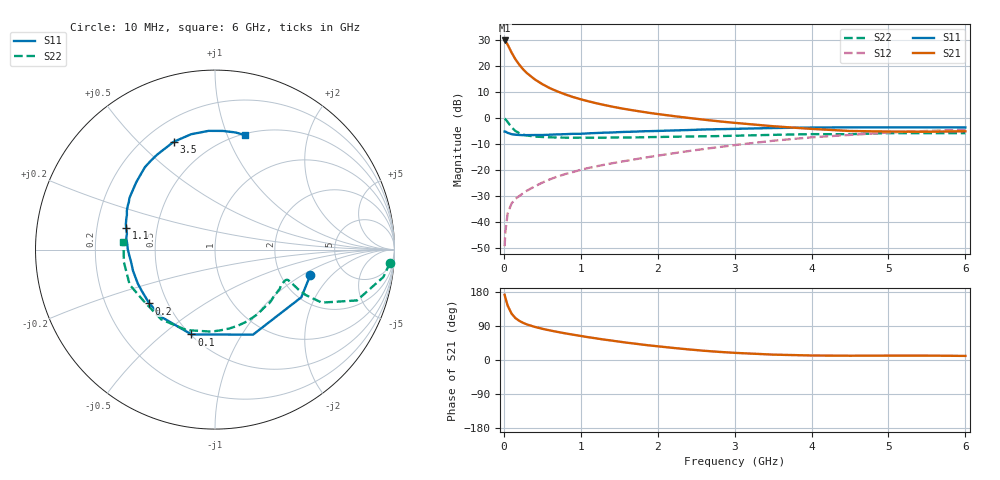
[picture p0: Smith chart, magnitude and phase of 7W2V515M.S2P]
! Infineon Technologies  Discrete & RF Semiconductors
! BFS17W
! Si NPN RF Bipolar Junction Transistor in SOT323
! VCE = 2.5 V  IC = 15 mA
! Common Emitter S-Parameters:  August  1999
# GHz  S  MA  R  50
!  f  S11  S21  S12  S22
! GHz  MAG  ANG  MAG  ANG  MAG  ANG  MAG  ANG
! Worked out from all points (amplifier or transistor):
!   36 points, 10 MHz to 6 GHz, reference 50 ohm
!   highest |S21| = 29.7 dB at 10 MHz (marker M1)
!   |S21| within 3 dB of that: start of sweep to 73.31 MHz
!   unconditionally stable (mu >= 1): 307.3 MHz to 2.534 GHz; 4.292 GHz to end of sweep
!   at 250 MHz: K = 0.93, MSG = 23.8 dB, |S12| = -28.8 dB
!   at 1.4 GHz: K = 1.21, MAG = 8.1 dB, |S12| = -17.4 dB
!   at 6 GHz: K = 1.08, MAG = -2.0 dB, |S12| = -4.4 dB
!   S11 on the Smith chart (normalised r, x): 10 MHz: 2.92, -1.18; 100 MHz: 0.51, -0.63; 200 MHz: 0.40, -0.31; 1.1 GHz: 0.33, +0.11; 3.5 GHz: 0.31, +0.64; 6 GHz: 0.52, +1.16
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0.01  0.55 -14.8  30.64 172.1  0.0035 81.5  0.9777 -4.3
0.02  0.5494 -28.9  29.83 163.8  0.0067 74.7  0.9499 -9.3
0.05  0.519 -65.9  25.45 143.4  0.0149 67.0  0.8401 -19.7
0.1  0.4906 -105.5  18.07 122.6  0.023 56.5  0.6644 -26.4
0.15  0.4788 -127.8  13.41 110.7  0.0283 54.8  0.565 -26.6
0.2  0.4733 -140.7  10.54 103.4  0.0319 56.8  0.5126 -25.5
0.25  0.4685 -149.9  8.61 98.1  0.0361 57.9  0.4804 -24.2
0.3  0.47 -156.2  7.264 93.9  0.0405 59.9  0.4634 -23.4
0.4  0.4718 -165.5  5.531 87.5  0.0488 62.2  0.4411 -22.6
0.5  0.4726 -171.7  4.458 82.4  0.0578 64.6  0.433 -22.8
0.6  0.4789 -176.2  3.724 78.0  0.0669 65.5  0.4268 -23.7
0.7  0.4857 179.9  3.218 74.0  0.0759 66.4  0.4231 -25.2
0.9  0.4984 172.8  2.523 66.8  0.0924 67.5  0.4189 -29.0
1.1  0.5085 166.5  2.088 60.1  0.1103 67.9  0.42 -33.7
1.3  0.5233 160.8  1.784 54.0  0.1266 68.1  0.4194 -39.2
1.6  0.5439 153.4  1.466 45.7  0.1519 68.4  0.4227 -47.6
2.2  0.5771 139.6  1.092 31.9  0.2105 68.0  0.438 -66.4
2.8  0.6108 125.8  0.863 21.4  0.2779 64.9  0.4509 -86.2
3.5  0.6432 111.0  0.696 14.2  0.3667 58.8  0.4758 -109.5
4.5  0.6625 93.1  0.564 11.3  0.4745 45.9  0.4892 -143.5
5.5  0.6626 80.1  0.546 11.6  0.5639 33.5  0.5123 -172.1
6  0.6598 75.1  0.557 10.8  0.5995 27.5  0.512 175.3
